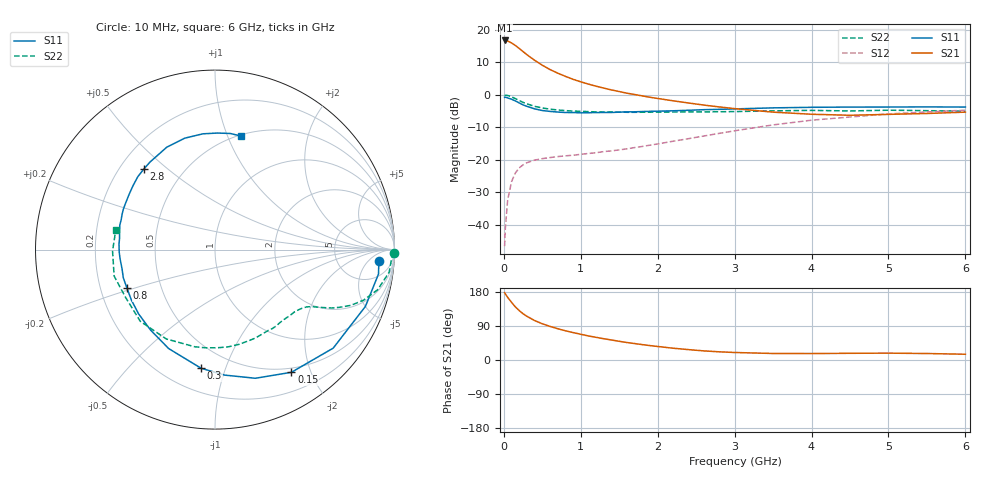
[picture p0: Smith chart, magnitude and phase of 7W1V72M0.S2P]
! Infineon Technologies  Discrete & RF Semiconductors
! BFS17W
! Si NPN RF Bipolar Junction Transistor in SOT323
! VCE = 1.75 V  IC = 2 mA
! Common Emitter S-Parameters:  August  1999
# GHz  S  MA  R  50
!  f  S11  S21  S12  S22
! GHz  MAG  ANG  MAG  ANG  MAG  ANG  MAG  ANG
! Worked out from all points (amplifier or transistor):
!   36 points, 10 MHz to 6 GHz, reference 50 ohm
!   highest |S21| = 16.7 dB at 10 MHz (marker M1)
!   |S21| within 3 dB of that: start of sweep to 227.5 MHz
!   unconditionally stable (mu >= 1): 792 MHz to end of sweep
!   at 250 MHz: K = 0.37, MSG = 17.4 dB, |S12| = -21.5 dB
!   at 1.4 GHz: K = 1.35, MAG = 5.9 dB, |S12| = -17.2 dB
!   at 6 GHz: K = 1.12, MAG = -2.4 dB, |S12| = -4.7 dB
!   S11 on the Smith chart (normalised r, x): 10 MHz: 14, -11; 150 MHz: 0.44, -1.71; 300 MHz: 0.35, -0.83; 800 MHz: 0.31, -0.19; 2.8 GHz: 0.30, +0.41; 6 GHz: 0.51, +1.11
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0.01  0.9152 -4.0  6.868 177.7  0.0047 84.9  0.9985 -1.0
0.02  0.9211 -8.5  6.831 174.2  0.0091 87.4  0.9851 -3.0
0.05  0.8958 -20.7  6.733 165.3  0.0243 78.9  0.9785 -7.4
0.1  0.8574 -39.8  6.286 152.2  0.0462 68.4  0.933 -13.9
0.15  0.8053 -58.1  5.752 140.1  0.0629 59.6  0.8744 -18.8
0.2  0.7512 -72.6  5.17 130.4  0.0752 53.6  0.8181 -22.3
0.25  0.7013 -85.6  4.624 122.1  0.0838 48.0  0.7662 -24.8
0.3  0.6655 -96.7  4.148 115.3  0.0903 44.6  0.7271 -26.6
0.4  0.6088 -115.1  3.402 104.1  0.0991 39.5  0.6658 -28.9
0.5  0.5743 -128.7  2.857 95.6  0.1044 37.2  0.6277 -30.4
0.6  0.5564 -139.9  2.45 88.6  0.1084 36.4  0.6025 -32.0
0.8  0.5352 -156.5  1.926 77.1  0.1152 37.2  0.5724 -36.0
0.9  0.5345 -162.9  1.735 72.4  0.1178 38.0  0.5626 -38.1
1.1  0.5312 -174.2  1.464 63.5  0.1253 40.8  0.5522 -42.9
1.3  0.5357 176.7  1.269 56.1  0.1341 43.8  0.5442 -48.4
1.6  0.5478 165.5  1.061 46.1  0.1477 48.3  0.5392 -56.9
2.2  0.5686 147.5  0.81 31.1  0.1933 55.7  0.5446 -75.8
2.8  0.5986 131.7  0.652 21.6  0.2554 57.6  0.5496 -95.6
3.5  0.6308 115.2  0.542 17.2  0.3451 54.2  0.567 -118.6
4.5  0.6486 96.0  0.485 17.7  0.4563 42.7  0.5649 -151.9
5.5  0.6526 82.5  0.517 17.1  0.546 30.8  0.5709 -179.3
6  0.6489 77.3  0.542 15.2  0.5807 25.2  0.5633 168.6
